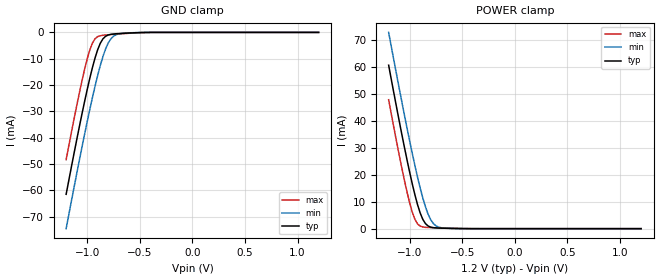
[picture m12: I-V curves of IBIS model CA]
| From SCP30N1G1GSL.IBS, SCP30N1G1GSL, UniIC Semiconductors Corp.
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|   Model CA
[Model] CA
Model_type Input
Vinl =  0.500V
Vinh =  0.700V
C_comp   1.051pF   1.012pF   1.102pF
[Model Spec]
Vinh   0.700V   0.670V   0.750V
Vinl   0.500V   0.470V   0.550V
[Temperature Range]   25.000   85.000   -40.000
[Voltage Range]   1.200V   1.140V   1.300V
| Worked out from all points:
|   GND clamp passes 1 mA (typ) near -0.80 V on its own axis
|   POWER clamp passes 1 mA (typ) near -0.83 V on its own axis
[GND_clamp]
|Voltage   I(typ)   I(min)   I(max)
-1.2V     -61.55mA   -74.61mA   -48.37mA
-1.05V    -31.07mA   -43.7mA    -18.49mA
-1V       -21.76mA   -33.97mA   -10.1mA
-975mV    -17.41mA   -29.28mA   -6.66mA
-925mV    -9.673mA   -20.4mA    -2.4mA
-875mV    -4.095mA   -12.51mA   -1.26mA
-850mV    -2.437mA   -9.132mA   -1.094mA
-800mV    -992.4uA   -4.024mA   -898.9uA
-750mV    -614.3uA   -1.442mA   -739.8uA
-675mV    -395.3uA   -396.9uA   -520.7uA
-500mV    -81.48uA   -51.49uA   -118.8uA
1.2V      0A         0A         0A
[POWER_clamp]
|Voltage   I(typ)   I(min)   I(max)
-1.2V     60.73mA    72.94mA    47.9mA
-1.125V   45.16mA    57.34mA    32.4mA
-1.05V    30.24mA    42.21mA    17.95mA
-1V       20.92mA    32.54mA    9.554mA
-950mV    12.52mA    23.39mA    3.432mA
-900mV    5.796mA    15.06mA    945.4uA
-850mV    1.867mA    8.09mA     492.9uA
-800mV    567.8uA    3.306mA    379uA
-750mV    278.4uA    1.047mA    302.5uA
-700mV    190.2uA    341.3uA    234.9uA
-550mV    61.32uA    49.14uA    76.57uA
1.2V      0A         0A         0A
